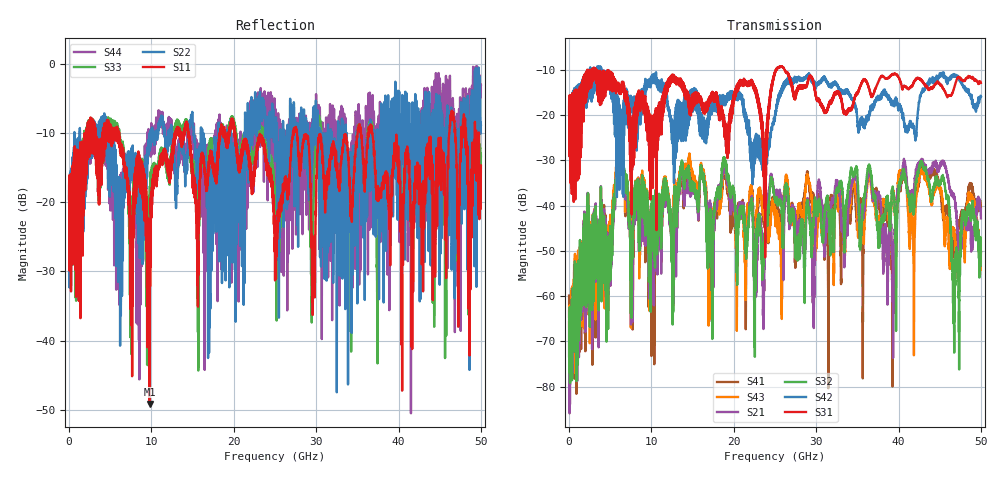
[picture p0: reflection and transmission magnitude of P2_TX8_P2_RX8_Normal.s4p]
!Keysight Technologies,N5225B,MY57041031,A.13.20.10
!Date: Friday, May 31, 2019 11:39:58
!Correction: S11(Full 4 Port(1,2,3,4))
!S12(Full 4 Port(1,2,3,4))
!S13(Full 4 Port(1,2,3,4))
!S14(Full 4 Port(1,2,3,4))
!S21(Full 4 Port(1,2,3,4))
!S22(Full 4 Port(1,2,3,4))
!S23(Full 4 Port(1,2,3,4))
!S24(Full 4 Port(1,2,3,4))
!S31(Full 4 Port(1,2,3,4))
!S32(Full 4 Port(1,2,3,4))
!S33(Full 4 Port(1,2,3,4))
!S34(Full 4 Port(1,2,3,4))
!S41(Full 4 Port(1,2,3,4))
!S42(Full 4 Port(1,2,3,4))
!S43(Full 4 Port(1,2,3,4))
!S44(Full 4 Port(1,2,3,4))
!S4P File: Measurements: <S11,S12,S13,S14>,
!<S21,S22,S23,S24>,
!<S31,S32,S33,S34>,
!<S41,S42,S43,S44>:
# Hz S  dB  R 50.0
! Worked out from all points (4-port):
!   5000 points, 10 MHz to 50 GHz, reference 50 ohm
!   strongest paths, dB at 10 MHz, 12.51 GHz, 25.01 GHz, 37.51 GHz, 50 GHz:
!     S31: -19.3, -11.7, -10.3, -12.8, -12.9
!     S42: -19.6, -21.4, -19.9, -16.1, -16.0
!     S32: -73.4, -47.2, -38.7, -46.4, -50.1
!     S21: -65.8, -48.3, -37.4, -37.5, -42.8
!     S43: -63.4, -48.6, -42.8, -43.3, -50.3
!     S41: -59.9, -50.0, -40.2, -37.8, -40.6
!   lowest |S11| = -49.2 dB at 9.79 GHz (marker M1), VSWR 1.01, Z = 50 - j0.346 ohm
!   |S11| at or under -10 dB: 20.17 GHz to 27.18 GHz (7.012 GHz wide, 29.6 % of centre); 27.67 GHz to 35.04 GHz (7.368 GHz wide, 23.5 % of centre); 36.81 GHz to 46.15 GHz (9.337 GHz wide, 22.5 % of centre)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
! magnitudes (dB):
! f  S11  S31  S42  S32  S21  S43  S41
! 10 MHz  -19.6  -19.3  -19.6  -73.4  -65.8  -63.4  -59.9
! 6.15 GHz  -12.1  -14.9  -30.5  -26.1  -26.7  -26.0  -26.6
! 9.79 GHz  -49.2  -26.2  -13.8  -44.5  -44.9  -45.5  -45.8
! 36.39 GHz  -9.9  -14.0  -20.5  -31.1  -32.2  -33.8  -32.8
! 39.41 GHz  -13.5  -11.0  -17.4  -37.6  -63.7  -37.2  -53.3
! 40.55 GHz  -26.5  -13.8  -19.5  -32.4  -31.3  -31.8  -33.3
! 50 GHz  -14.7  -12.9  -16.0  -50.1  -42.8  -50.3  -40.6
